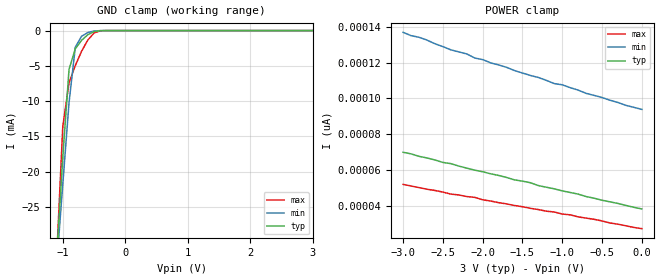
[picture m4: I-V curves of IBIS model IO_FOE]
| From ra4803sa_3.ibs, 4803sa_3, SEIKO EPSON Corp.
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[Model]   IO_FOE
Model_type Input
Enable Active-High
Polarity Non-Inverting
Vinh=2.4
Vinl=0.6
C_comp   5p   4p   6p
[Temperature Range] 25   85   -40
[Voltage Range]   3.0   2.7   3.3
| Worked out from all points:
|   GND clamp passes 1 mA (typ) near -0.65 V on its own axis
[GND Clamp]
-3V       -321.4mA   -266.3mA   -408.9mA
-1.1V     -32.43mA   -33.46mA   -32.61mA
-1V       -17.96mA   -21.79mA   -13.59mA
-900mV    -5.499mA   -10.22mA   -7.421mA
-800mV    -2.576mA   -2.362mA   -4.965mA
-700mV    -1.392mA   -807.3uA   -2.943mA
-600mV    -591.5uA   -281.9uA   -1.347mA
-500mV    -144.6uA   -61.93uA   -343.6uA
-400mV    -15.25uA   -7.313uA   -28.72uA
3V        38.09pA    97.66pA    24.56pA
[POWER Clamp]
-3V       69.8pA     136.9pA    51.84pA
-2.7V     66.62pA    132.6pA    49.11pA
-2.4V     63.44pA    127.1pA    46.38pA
-2.2V     60.94pA    124.8pA    45.02pA
-2.1V     59.8pA     122.6pA    44.57pA
-2V       58.89pA    121.6pA    43.2pA
-1.4V     52.75pA    112.8pA    38.43pA
-1.3V     51.16pA    111.6pA    37.74pA
-1.1V     49.34pA    108.2pA    36.38pA
-1V       48.2pA     107.5pA    35.24pA
-700mV    45.02pA    102.8pA    32.97pA
0V        38.09pA    93.79pA    27.06pA
